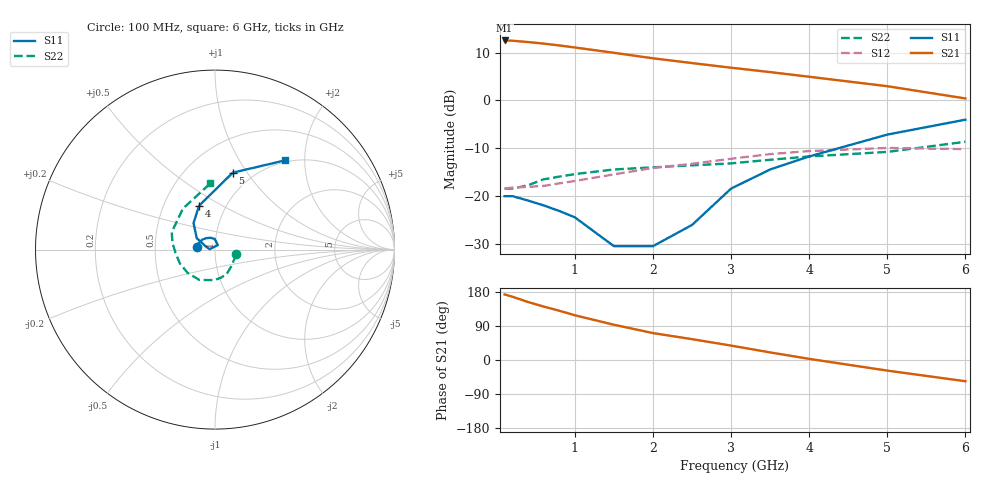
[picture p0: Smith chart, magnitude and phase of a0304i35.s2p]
!  MSA-0304 S AND NOISE PARAMETERS
!  Id=35mA  LAST UPDATED 07-22-92
# ghz s ma r 50
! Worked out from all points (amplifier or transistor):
!   14 points, 100 MHz to 6 GHz, reference 50 ohm
!   highest |S21| = 12.5 dB at 100 MHz (marker M1)
!   |S21| within 3 dB of that: start of sweep to 1.682 GHz
!   unconditionally stable (mu >= 1): start of sweep to end of sweep
!   at 400 MHz: K = 1.21, MAG = 12.4 dB, |S12| = -18.1 dB
!   at 2 GHz: K = 1.15, MAG = 9.1 dB, |S12| = -14.1 dB
!   at 6 GHz: K = 1.10, MAG = 3.3 dB, |S12| = -10.2 dB
!   lowest NFmin = 5.60 dB at 100 MHz
!   S11 on the Smith chart (normalised r, x): 100 MHz: 0.82, +0.02; 4 GHz: 0.75, +0.39; 5 GHz: 0.81, +0.86; 6 GHz: 0.97, +1.60
0.1  0.1 173.0  4.24 173.0  0.12 3.0  0.12 -13.0
0.2  0.1 162.0  4.21 167.0  0.123 4.0  0.12 -24.0
0.4  0.09 142.0  4.08 153.0  0.125 7.0  0.13 -46.0
0.6  0.08 127.0  3.93 141.0  0.128 10.0  0.15 -64.0
0.8  0.07 110.0  3.76 130.0  0.136 14.0  0.16 -78.0
1  0.06 92.0  3.58 118.0  0.144 16.0  0.17 -91.0
1.5  0.03 58.0  3.15 93.0  0.169 19.0  0.19 -117.0
2  0.03 175.0  2.76 71.0  0.197 18.0  0.2 -139.0
2.5  0.05 163.0  2.46 55.0  0.218 18.0  0.21 -158.0
3  0.12 148.0  2.2 38.0  0.246 15.0  0.22 -174.0
3.5  0.19 129.0  1.98 20.0  0.275 7.0  0.24 171.0
4  0.26 110.0  1.77 3.0  0.296 1.0  0.26 158.0
5  0.44 77.0  1.41 -28.0  0.319 -15.0  0.29 128.0
6  0.63 52.0  1.05 -56.0  0.31 -31.0  0.37 94.0
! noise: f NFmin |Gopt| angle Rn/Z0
0.1  5.6  0.05  1  0.86
0.5  5.8  0.05  8  0.86
1  6  0.04  0  0.85
2  6.5  0.02  -69  0.82
